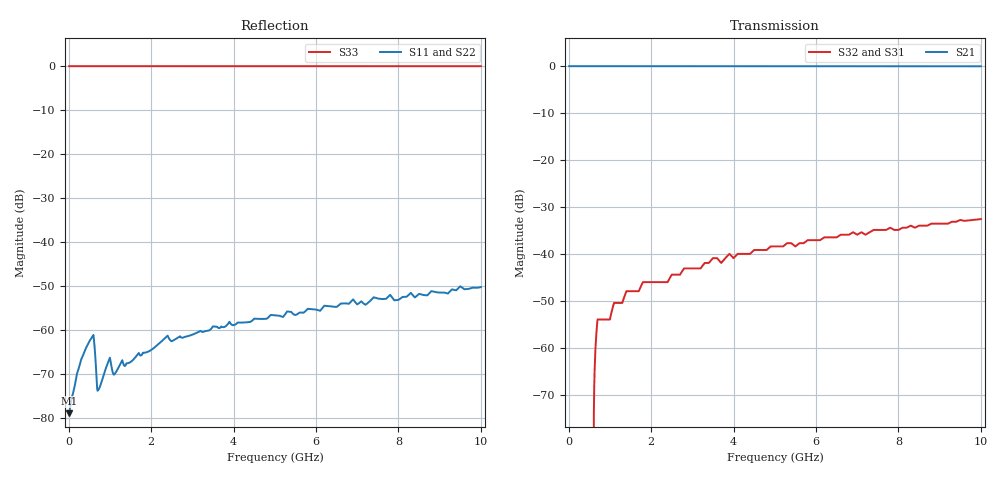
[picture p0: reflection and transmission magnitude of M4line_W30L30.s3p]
! Created Fri Sep 09 14:15:09 2011
# hz S ma R 50
! 3 Port Network Data from SP1.SP block
! freq  magS11  angS11  magS12  angS12  magS13  angS13
!  magS21  angS21
!  magS22  angS22  magS23  angS23
!  magS31  angS31  magS32  angS32
!  magS33  angS33
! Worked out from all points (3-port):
!   1000 points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, 10 MHz to 10 GHz, reference 50 ohm
!   strongest paths, dB at 10 MHz, 2.51 GHz, 5.01 GHz, 7.51 GHz, 10 GHz:
!     S21: 0.0, 0.0, 0.0, 0.0, 0.0
!     S32: -, -44.4, -38.4, -34.9, -32.6
!     S31: -, -44.4, -38.4, -34.9, -32.6
!   lowest |S11| = -79.0 dB at 10 MHz (marker M1), VSWR 1.00, Z = 50 + j0.00148 ohm
!   |S11| at or under -10 dB: start of sweep to end of sweep
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1e7  0.0001119 7.6  0.9999 -0.0  0 0.0
     0.9999 -0.0  0.0001119 7.6  0 0.0
     0 0.0  0 0.0  1 0.0
5.5e8  0.0008004 77.6  0.9998 -0.0  0 0.0
       0.9998 -0.0  0.0008004 77.6  0 0.0
       0 0.0  0 0.0  1 0.0
5.9e8  0.0008573 77.9  0.9998 -0.0  0 0.0
       0.9998 -0.0  0.0008573 77.9  0 0.0
       0 0.0  0 0.0  1 0.0
6.7e8  0.0003154 51.5  0.9998 -0.1  0.0014 89.9
       0.9998 -0.1  0.0003154 51.5  0.0014 89.9
       0.0014 89.9  0.0014 89.9  1 -0.2
7.2e8  0.0002072 4.8  0.9998 -0.1  0.002 89.8
       0.9998 -0.1  0.0002072 4.8  0.002 89.8
       0.002 89.8  0.002 89.8  1 -0.2
9.7e8  0.0004424 51.9  0.9997 -0.1  0.002 89.8
       0.9997 -0.1  0.0004424 51.9  0.002 89.8
       0.002 89.8  0.002 89.8  1 -0.2
1.42e9  0.000415 -13.8  0.9996 -0.2  0.004 89.7
        0.9996 -0.2  0.000415 -13.8  0.004 89.7
        0.004 89.7  0.004 89.7  1 -0.5
2.37e9  0.0008305 32.0  0.9993 -0.3  0.005 89.6
        0.9993 -0.3  0.0008305 32.0  0.005 89.6
        0.005 89.6  0.005 89.6  1 -0.6
5.01e9  0.001458 -22.7  0.9985 -0.7  0.012 89.0
        0.9985 -0.7  0.001458 -22.7  0.012 89.0
        0.012 89.0  0.012 89.0  0.9999 -1.4
1e10  0.003056 -43.2  0.9971 -1.2  0.02348 87.7
      0.9971 -1.2  0.003056 -43.2  0.02348 87.7
      0.02348 87.7  0.02348 87.7  0.9992 -2.7
